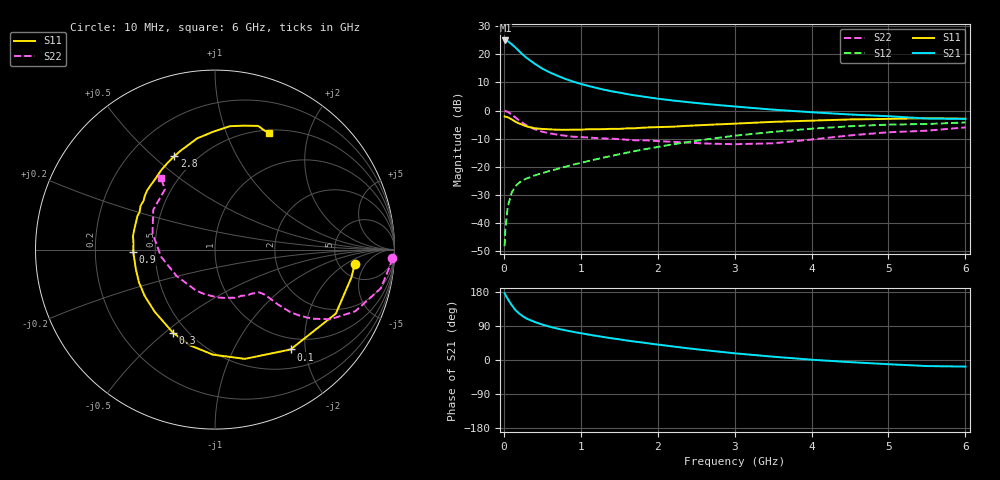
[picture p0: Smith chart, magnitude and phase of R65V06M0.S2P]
! SIEMENS Small Signal Semiconductors
! BFR193
! Si NPN RF Bipolar Junction Transistor in SOT23
! VCE = 5 V  IC = 6 mA
! Common Emitter S-Parameters:  May  1996
# GHz  S  MA  R  50
!  f  S11  S21  S12  S22
! GHz  MAG  ANG  MAG  ANG  MAG  ANG  MAG  ANG
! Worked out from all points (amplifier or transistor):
!   36 points, 10 MHz to 6 GHz, reference 50 ohm
!   highest |S21| = 25.0 dB at 20 MHz (marker M1)
!   |S21| within 3 dB of that: start of sweep to 168.4 MHz
!   unconditionally stable (mu >= 1): 870.5 MHz to 2.01 GHz
!   at 250 MHz: K = 0.47, MSG = 22.3 dB, |S12| = -24.8 dB
!   at 1.4 GHz: K = 1.05, MAG = 10.1 dB, |S12| = -16.2 dB
!   at 6 GHz: K = 0.96, MSG = 0.6 dB, |S12| = -4.3 dB
!   lowest NFmin = 1.20 dB at 450 MHz
!   S11 on the Smith chart (normalised r, x): 10 MHz: 7.07, -2.85; 100 MHz: 0.80, -1.73; 300 MHz: 0.42, -0.53; 900 MHz: 0.37, -0.01; 2.8 GHz: 0.38, +0.59; 6 GHz: 0.54, +1.42
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0.01  0.7836 -5.7  17.66 176.4  0.0038 87.3  0.9882 -2.7
0.02  0.7758 -11.5  17.78 172.2  0.0077 85.0  0.9792 -5.4
0.05  0.7619 -27.9  17.3 161.3  0.0189 76.0  0.9482 -13.2
0.1  0.6977 -52.9  15.32 145.6  0.0338 65.8  0.854 -23.7
0.15  0.6311 -74.7  13.31 131.9  0.0445 58.4  0.7513 -31.1
0.2  0.5854 -91.2  11.44 122.6  0.0517 54.0  0.663 -35.5
0.25  0.5508 -104.8  9.818 115.0  0.0574 51.4  0.5946 -38.1
0.3  0.5186 -116.9  8.616 109.0  0.0615 50.1  0.5395 -39.8
0.4  0.4825 -134.1  6.852 100.4  0.0695 50.0  0.4641 -41.1
0.5  0.4694 -146.6  5.584 93.5  0.0763 50.9  0.4189 -41.5
0.6  0.4611 -156.8  4.763 87.7  0.0838 52.3  0.3912 -41.8
0.7  0.4547 -165.4  4.154 82.7  0.091 53.7  0.3699 -42.4
0.9  0.4556 -178.5  3.283 74.3  0.1082 56.7  0.3414 -44.2
1.1  0.4632 170.7  2.741 67.1  0.1257 58.3  0.3296 -47.4
1.3  0.4656 161.1  2.355 60.5  0.145 59.3  0.3173 -51.1
1.6  0.4806 149.7  1.965 51.4  0.1769 59.7  0.3013 -58.4
2.2  0.515 130.3  1.506 35.7  0.2496 56.6  0.2762 -77.6
2.8  0.5673 113.6  1.245 22.0  0.3276 50.2  0.2541 -104.8
3.5  0.6278 99.1  1.036 8.7  0.4157 39.8  0.2596 -145.6
4.5  0.6927 83.1  0.849 -5.6  0.5245 23.7  0.3597 165.3
5.5  0.7297 70.8  0.719 -16.0  0.5743 6.9  0.4365 129.7
6  0.713 65.2  0.708 -17.4  0.613 2.1  0.4994 127.1
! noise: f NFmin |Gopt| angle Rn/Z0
0.45  1.2  0.25  114  0.13
0.9  1.25  0.37  150  0.12
1.8  2  0.55  -158  0.12
